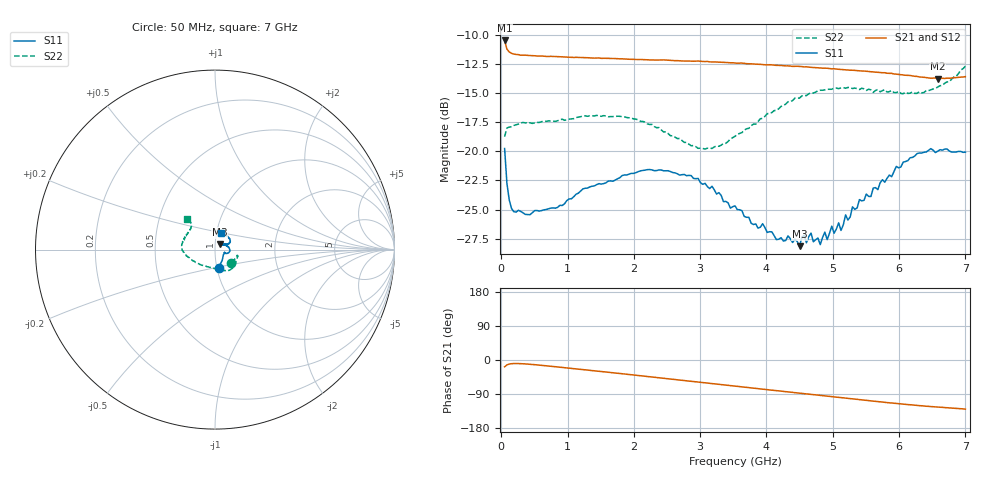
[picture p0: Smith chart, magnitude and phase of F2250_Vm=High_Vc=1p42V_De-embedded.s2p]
! Integrated Device Technology
! Corporate Headquarters
! 6024 Silver Creek Valley Road
! San Jose, CA 95138  USA
! Phone:  1-408-284-8200
! Toll Free:  1-800-223-1366
! Webpage:  http://www.idt.com/
! Timing and RF Division
! 515 Groton Road, Suite 102
! Westford, MA 01886-6024
! Device:  F2250
! Description: Voltage Variable RF Attenuator
! Frequency:  50.0 -  6000.00 MHz
! Package:  3x3 mm Thin QFN Plastic Package: 16 pin
! Ports:  2 RF, 3 DC
!  Pin  1  = GND
!  Pin  2  = NC
!  Pin  3  = RF1  = Port 1
!  Pin  4  = NC
!  Pin  5  = GND
!  Pin  6  = GND
!  Pin  7  = GND
!  Pin  8  = GND
!  Pin  9  = NC
!  Pin 10  = RF2  = Port 2
!  Pin 11  = NC
!  Pin 12  = GND
!  Pin 13  = GND
!  Pin 14  = VCNTRL
!  Pin 15  = VDD
!  Pin 16  = VMODE
! Vcntrl:  1.420 Volts
! Vmode:  +3.300 Volts
! Vdd:  +3.30  Volts
! Current:  1.328 mA
! Data:  The device was measured on a the F2250 evaluation board which has
!  individual transmission lines to the RF pins.  Data was collected
!  using a calibrated network analyzer.  The evaluation board was
!  de-embedded using a TRL calibration technique.
!  The reference plane is the edge of the package pin.
! Misc:  SN 10
!  Action Tracker AT0258
! Date Measured:  2014-11-26
! Date:  2015-10-15  MJV
! Note:
!  Integrated Device Technology supplies this data as a sample of measured
!  data at the package pin for this product.  Your particular data for this
!  product may vary.
!  Data was taken at 25 degrees C.
!  Integrated Device Technology reserves the right to change this data at anytime.
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# GHz S dB R 50
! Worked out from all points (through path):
!   201 points, 50 MHz to 7 GHz, reference 50 ohm
!   highest |S21| = -10.50 dB at 50 MHz (marker M1); lowest = -13.8 dB at 6.583 GHz (marker M2)
!   group delay of S21, straight-line fit = 51.3 ps
!   lowest |S11| = -28.1 dB at 4.498 GHz (marker M3), VSWR 1.08, Z = 52.5 + j3.11 ohm
!   |S11| at or under -10 dB: start of sweep to end of sweep
!   |S22| runs from -19.8 to -12.7 dB; largest |S21 - S12| = 0.0015
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0.05  -19.77 -79.0  -10.50 -17.9  -10.50 -17.9  -18.75 -38.7
0.08475  -22.75 -56.7  -11.24 -12.9  -11.25 -12.9  -18.01 -21.4
0.1195  -24.17 -45.6  -11.48 -10.7  -11.50 -10.7  -17.93 -16.2
0.189  -25.19 -32.0  -11.66 -9.3  -11.66 -9.3  -17.79 -14.3
0.8145  -24.88 -16.5  -11.87 -17.7  -11.90 -17.7  -17.43 -29.8
1.2315  -23.23 -18.1  -11.95 -25.3  -11.97 -25.4  -16.97 -41.4
2.37825  -21.60 -2.4  -12.18 -46.7  -12.19 -46.7  -17.97 -67.9
2.969  -22.33 12.1  -12.26 -58.1  -12.29 -58.1  -19.75 -96.2
3.525  -24.69 28.8  -12.43 -68.9  -12.43 -68.9  -18.72 -133.2
3.8725  -26.60 41.4  -12.54 -75.5  -12.54 -75.5  -17.45 -151.5
4.498  -28.14 49.1  -12.72 -87.6  -12.74 -87.6  -15.44 -172.2
4.5675  -27.20 51.1  -12.77 -88.9  -12.76 -88.9  -15.22 -173.4
4.7065  -27.77 51.6  -12.82 -91.6  -12.81 -91.6  -15.01 -176.6
4.81075  -28.01 46.6  -12.86 -93.5  -12.86 -93.5  -14.77 -178.6
4.88025  -26.94 44.6  -12.88 -94.9  -12.86 -94.9  -14.73 179.3
4.915  -27.58 43.8  -12.88 -95.6  -12.89 -95.5  -14.69 178.5
5.08875  -26.14 38.4  -12.97 -98.8  -12.97 -98.9  -14.63 174.7
5.1235  -26.79 38.0  -12.98 -99.5  -12.97 -99.5  -14.57 173.8
5.29725  -24.77 29.3  -13.05 -102.7  -13.03 -102.8  -14.62 170.3
5.85325  -22.04 23.4  -13.32 -112.9  -13.30 -113.1  -14.89 155.2
6.583  -19.99 39.3  -13.76 -124.1  -13.76 -124.3  -14.48 133.8
7  -20.08 69.5  -13.60 -129.5  -13.61 -129.7  -12.71 132.6
